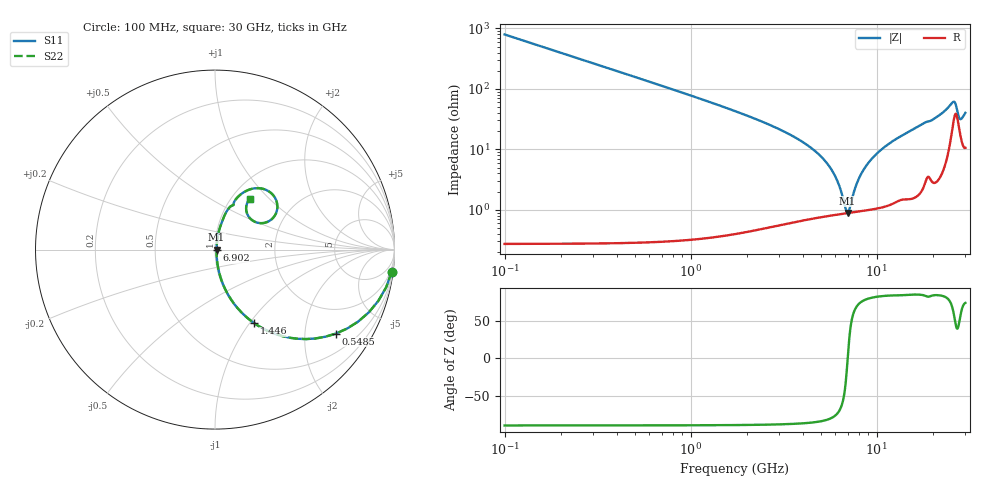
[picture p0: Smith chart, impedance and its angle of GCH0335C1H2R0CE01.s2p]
!Murata Part Number: GCH0335C1H2R0CE01
!These Parameters are Measured in Series Mode Connection
!Data Generated on Jun 19, 2026
!  o--ll--o
!Port1  Port2
!  o------o
!Operation Temp=25[degC], DC Bias Voltage=0[V]
!Freq. Start=100[MHz] Stop=30[GHz] 401[Steps]
# Hz S RI R 50
!Freq.(Hz) S11(Real) S11(Imag) S21(Real) S21(Imag) S12(Real) S12(Imag) S22(Real) S22(Imag)
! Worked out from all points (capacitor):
!   401 points, 100 MHz to 30 GHz, reference 50 ohm
!   read as one part in series: C = 2 pF near 249.5 MHz
!   lowest |Z| = 881 mohm at 6.977 GHz (marker M1)
!   series resonance near 6.987 GHz, so ESL is about 260 pH
!   S11 on the Smith chart (normalised r, x): 100 MHz: 1, -16; 548.5 MHz: 1.01, -2.88; 1.446 GHz: 1.01, -1.05; 6.902 GHz: 1.02, -0.01; 30 GHz: 1.21, +0.77
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1e8  0.9844 -0.1237  0.0156 0.1237  0.0156 0.1237  0.9844 -0.1237
3.2425e8  0.8568 -0.3497  0.1432 0.3497  0.1432 0.3497  0.8568 -0.3497
5.485e8  0.6747 -0.4675  0.3253 0.4675  0.3253 0.4675  0.6747 -0.4675
9.97e8  0.3792 -0.4832  0.6208 0.4832  0.6208 0.4832  0.3792 -0.4832
1.4455e9  0.218 -0.4094  0.782 0.4094  0.782 0.4094  0.218 -0.4094
2.6415e9  0.0658 -0.2383  0.9342 0.2383  0.9342 0.2383  0.0658 -0.2383
5.10825e9  0.0125 -0.0703  0.9875 0.0703  0.9875 0.0703  0.0125 -0.0703
6.08e9  0.00917 -0.0309  0.9908 0.0309  0.9908 0.0309  0.00917 -0.0309
6.90225e9  0.00869 -0.0027  0.9913 0.0027  0.9913 0.0027  0.00869 -0.0027
6.977e9  0.00872 -0.000307  0.9913 0.000307  0.9913 0.000307  0.00872 -0.000307
7.1265e9  0.00882 0.0044  0.9912 -0.0044  0.9912 -0.0044  0.00882 0.0044
7.7245e9  0.00962 0.0223  0.9904 -0.0223  0.9904 -0.0223  0.00962 0.0223
8.24775e9  0.0108 0.037  0.9892 -0.037  0.9892 -0.037  0.0108 0.037
1.01165e10  0.0176 0.0842  0.9824 -0.0842  0.9824 -0.0842  0.0176 0.0842
1.22095e10  0.03 0.1305  0.97 -0.1305  0.97 -0.1305  0.03 0.1305
1.505e10  0.051 0.1856  0.949 -0.1856  0.949 -0.1856  0.051 0.1856
2.005825e10  0.1083 0.2686  0.8917 -0.2686  0.8917 -0.2686  0.1083 0.2686
2.50665e10  0.2862 0.3319  0.7138 -0.3319  0.7138 -0.3319  0.2862 0.3319
2.62625e10  0.3473 0.2337  0.6527 -0.2337  0.6527 -0.2337  0.3473 0.2337
2.7309e10  0.2606 0.1473  0.7394 -0.1473  0.7394 -0.1473  0.2606 0.1473
2.8206e10  0.1869 0.1849  0.8131 -0.1849  0.8131 -0.1849  0.1869 0.1849
3e10  0.1944 0.2821  0.8056 -0.2821  0.8056 -0.2821  0.1944 0.2821
